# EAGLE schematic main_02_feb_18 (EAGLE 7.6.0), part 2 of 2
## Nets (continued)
Unconnected: IC1.11(CLK) IC1.18(8D) IC2.1(A:G) IC2.2(A:A1) IC2.4(A:A2) IC2.6(A:A3) IC2.8(A:A4) IC2.12(A:Y4) IC2.14(A:Y3) IC2.16(A:Y2) IC2.18(A:Y1) IC3.1(A:G) IC3.2(A:A1) IC3.4(A:A2) IC3.6(A:A3) IC3.8(A:A4) IC3.12(A:Y4) IC3.14(A:Y3) IC3.16(A:Y2) IC3.18(A:Y1) IC4.11(CLK) IC5.11(CLK) IC6.4(2D) IC6.7(3D) IC6.8(4D) IC6.11(CLK) IC6.13(5D) IC6.14(6D) IC6.17(7D) IC7.4(2D) IC7.7(3D) IC7.8(4D) IC7.13(5D) IC7.14(6D) IC7.17(7D) IC8.1(A:G) IC8.2(A:A1) IC8.4(A:A2) IC8.6(A:A3) IC8.8(A:A4) IC8.12(A:Y4) IC8.14(A:Y3) IC8.16(A:Y2) IC8.18(A:Y1) IC10.3(B:Y4) IC10.5(B:Y3) IC10.7(B:Y2) IC10.9(B:Y1) IC10.11(B:A1) IC10.13(B:A2) IC10.15(B:A3) IC10.17(B:A4) IC10.19(B:G) IC11.3(B:Y4) IC11.5(B:Y3) IC11.7(B:Y2) IC11.9(B:Y1) IC11.11(B:A1) IC11.13(B:A2) IC11.15(B:A3) IC11.17(B:A4) IC11.19(B:G) IC12.3(B:Y4) IC12.5(B:Y3) IC12.7(B:Y2) IC12.9(B:Y1) IC12.11(B:A1) IC12.13(B:A2) IC12.15(B:A3) IC12.17(B:A4) IC12.19(B:G) IC13.3(B:Y4) IC13.5(B:Y3) IC13.7(B:Y2) IC13.9(B:Y1) IC13.11(B:A1) IC13.13(B:A2) IC13.15(B:A3) IC13.17(B:A4) IC13.19(B:G) IC14.14(A=B) IC14.15(P) IC14.17(G) IC15.14(A=B) IC15.15(P) IC15.17(G) IC16.11(CLK) IC17.11(CLK) IC18.1(A:I0) IC18.2(A:I1) IC18.3(A:O) IC18.8(C:O) IC18.9(C:I0) IC18.10(C:I1) IC18.11(D:O) IC18.12(D:I0) IC18.13(D:I1) IC19.2(A:A1) IC19.4(A:A2) IC19.6(A:A3) IC19.8(A:A4) IC19.11(B:A1) IC19.13(B:A2) IC19.15(B:A3) IC19.17(B:A4) IC20.5(Q2) IC20.6(Q3) IC20.9(Q4) IC20.11(CLK) IC20.12(Q5) IC20.15(Q6) IC20.16(Q7) IC21.11(CLK) IC24.1(A:G) IC24.2(A:A1) IC24.4(A:A2) IC24.6(A:A3) IC24.8(A:A4) IC24.12(A:Y4) IC24.14(A:Y3) IC24.16(A:Y2) IC24.18(A:Y1) IC25.1(A:G) IC25.2(A:A1) IC25.4(A:A2) IC25.6(A:A3) IC25.8(A:A4) IC25.12(A:Y4) IC25.14(A:Y3) IC25.16(A:Y2) IC25.18(A:Y1) IC26.1(A:G) IC26.2(A:A1) IC26.4(A:A2) IC26.6(A:A3) IC26.8(A:A4) IC26.12(A:Y4) IC26.14(A:Y3) IC26.16(A:Y2) IC26.18(A:Y1) IC27.1(A:G) IC27.2(A:A1) IC27.4(A:A2) IC27.6(A:A3) IC27.8(A:A4) IC27.12(A:Y4) IC27.14(A:Y3) IC27.16(A:Y2) IC27.18(A:Y1) IC28.1(A:G) IC28.2(A:A1) IC28.4(A:A2) IC28.6(A:A3) IC28.8(A:A4) IC28.12(A:Y4) IC28.14(A:Y3) IC28.16(A:Y2) IC28.18(A:Y1) IC29.1(A:G) IC29.2(A:A1) IC29.4(A:A2) IC29.6(A:A3) IC29.8(A:A4) IC29.12(A:Y4) IC29.14(A:Y3) IC29.16(A:Y2) IC29.18(A:Y1) IC30.3(B:Y4) IC30.5(B:Y3) IC30.7(B:Y2) IC30.9(B:Y1) IC30.11(B:A1) IC30.13(B:A2) IC30.15(B:A3) IC30.17(B:A4) IC30.19(B:G) IC31.3(B:Y4) IC31.5(B:Y3) IC31.7(B:Y2) IC31.9(B:Y1) IC31.11(B:A1) IC31.13(B:A2) IC31.15(B:A3) IC31.17(B:A4) IC31.19(B:G) IC32.17(D7) IC32.18(D8) IC33.16(Q7) IC33.19(Q8) IC34.1(1G) IC34.15(2G) IC35.1(1G) IC35.15(2G) IC36.1(1G) IC36.15(2G) IC37.1(1G) IC37.15(2G) IC38.1(1G) IC38.15(2G) IC39.4(B:I0) IC39.5(B:I1) IC39.6(B:O) IC39.8(C:O) IC39.9(C:I0) IC39.10(C:I1) IC39.11(D:O) IC39.12(D:I0) IC39.13(D:I1) IC40.1(1G) IC40.15(2G) IC41.1(1G) IC41.15(2G) IC42.4(B:I0) IC42.5(B:I1) IC42.6(B:O) IC42.8(C:O) IC42.9(C:I0) IC42.10(C:I1) IC42.11(D:O) IC42.12(D:I0) IC42.13(D:I1) IC43.1(A:I) IC43.2(A:O) IC43.5(C:I) IC43.6(C:O) IC43.8(D:O) IC43.9(D:I) IC43.10(E:O) IC43.11(E:I) IC43.12(F:O) IC43.13(F:I) IC44.6(A:!Q) IC44.8(B:!Q) IC44.9(B:Q) IC44.10(B:PRE) IC44.11(B:CLK) IC44.12(B:D) IC44.13(B:CLR) IC45.4(B:I0) IC45.5(B:I1) IC45.6(B:O) IC45.8(C:O) IC45.9(C:I0) IC45.10(C:I1) IC45.11(D:O) IC45.12(D:I0) IC45.13(D:I1) IC46.1(G) IC46.11(CLK) IC48.4(2D) IC48.7(3D) IC48.8(4D) IC48.11(CLK) IC48.13(5D) IC48.14(6D) IC48.17(7D) IC49.3(1B) IC49.6(2B) IC49.10(3B) IC49.13(4B) IC50.1(S2) IC50.10(S4) IC50.13(S3) IC51.1(S2) IC51.4(S1) IC51.10(S4) IC51.13(S3) IC52.1(S2) IC52.4(S1) IC52.10(S4) IC52.13(S3) IC53.4(S1) IC53.9(C4) IC53.10(S4) IC53.13(S3) IC54.1(A:I) IC54.2(A:O) IC54.5(C:I) IC54.6(C:O) IC54.8(D:O) IC54.9(D:I) IC54.10(E:O) IC54.11(E:I) IC54.12(F:O) IC54.13(F:I) IC55.3(1B) IC55.6(2B) IC55.10(3B) IC56.9(2Y) IC56.10(2C0) IC56.11(2C1) IC56.12(2C2) IC56.13(2C3) IC57.5(C:I) IC57.6(C:O) IC57.8(D:O) IC57.9(D:I) IC57.10(E:O) IC57.11(E:I) IC57.12(F:O) IC57.13(F:I) IC58.4(B:I0) IC58.5(B:I1) IC58.6(B:O) IC58.8(C:O) IC58.9(C:I0) IC58.10(C:I1) IC58.11(D:O) IC58.12(D:I0) IC58.13(D:I1) IC60.1(CLR) IC60.9(Q4) IC60.12(Q5) IC60.15(Q6) IC60.16(Q7) IC60.19(Q8) IC61.1(CLR) IC61.2(Q1) IC61.5(Q2) IC61.6(Q3) IC61.9(Q4) IC61.12(Q5) IC61.15(Q6) IC61.16(Q7) IC61.19(Q8) IC62.1(CLR) IC62.2(Q1) IC62.5(Q2) IC62.6(Q3) IC62.9(Q4) IC62.12(Q5) IC62.15(Q6) IC62.16(Q7) IC62.19(Q8) IC64.8(B:O) IC64.9(B:I0) IC64.10(B:I1) IC64.12(B:I2) IC64.13(B:I3) IC65.3(B:I) IC65.4(B:O) IC65.5(C:I) IC65.6(C:O) IC65.8(D:O) IC65.9(D:I) IC65.10(E:O) IC65.11(E:I) IC65.12(F:O) IC65.13(F:I) IC66.1(A:I0) IC66.2(A:I1) IC66.3(A:O) IC66.8(C:O) IC66.9(C:I0) IC66.10(C:I1) IC66.11(D:O) IC66.12(D:I0) IC66.13(D:I1) IC67.1(A:I0) IC67.2(A:I1) IC67.3(A:O) IC67.8(C:O) IC67.9(C:I0) IC67.10(C:I1) IC67.11(D:O) IC67.12(D:I0) IC67.13(D:I1) IC68.9(3Y) IC68.12(4Y) IC69.1(A:G) IC69.2(A:A1) IC69.3(B:Y4) IC69.4(A:A2) IC69.6(A:A3) IC69.8(A:A4) IC69.12(A:Y4) IC69.14(A:Y3) IC69.15(B:A3) IC69.16(A:Y2) IC69.18(A:Y1) IC70.1(A:G) IC70.2(A:A1) IC70.4(A:A2) IC70.6(A:A3) IC70.8(A:A4) IC70.12(A:Y4) IC70.14(A:Y3) IC70.16(A:Y2) IC70.18(A:Y1) IC71.1(A:G) IC71.2(A:A1) IC71.4(A:A2) IC71.6(A:A3) IC71.8(A:A4) IC71.12(A:Y4) IC71.14(A:Y3) IC71.16(A:Y2) IC71.18(A:Y1) IC72.1(A:I0) IC72.2(A:I1) IC72.3(A:O) IC72.8(C:O) IC72.9(C:I0) IC72.10(C:I1) IC72.11(D:O) IC72.12(D:I0) IC72.13(D:I1) IC73.5(2A) IC73.6(2B) IC73.7(2Y) IC73.9(3Y) IC73.10(3B) IC73.11(3A) IC73.12(4Y) IC73.13(4B) IC73.14(4A) IC73.15(G) IC74.1(A:I0) IC74.2(A:I1) IC74.3(A:O) IC74.8(C:O) IC74.9(C:I0) IC74.10(C:I1) IC74.11(D:O) IC74.12(D:I0) IC74.13(D:I1) IC75.2(Q1) IC75.5(Q2) IC75.6(Q3) IC75.9(Q4) IC75.12(Q5) IC75.15(Q6) IC75.16(Q7) IC75.19(Q8) IC76.2(Q1) IC77.2(Q1) IC80.1(A:I0) IC80.2(A:I1) IC80.3(A:O) IC80.8(C:O) IC80.9(C:I0) IC80.10(C:I1) IC80.11(D:O) IC80.12(D:I0) IC80.13(D:I1) IC81.1(A:I0) IC81.2(A:I1) IC81.3(A:O) IC81.8(C:O) IC81.9(C:I0) IC81.10(C:I1) IC81.11(D:O) IC81.12(D:I0) IC81.13(D:I1) IC82.11(CLK) IC83.1(A:I) IC83.2(A:O) IC83.5(C:I) IC83.6(C:O) IC83.8(D:O) IC83.9(D:I) IC83.10(E:O) IC83.11(E:I) IC83.12(F:O) IC83.13(F:I) IC84.1(A:I) IC84.2(A:O) IC84.5(C:I) IC84.6(C:O) IC84.8(D:O) IC84.9(D:I) IC84.10(E:O) IC84.11(E:I) IC84.12(F:O) IC84.13(F:I) IC85.1(A:I0) IC85.2(A:I1) IC85.3(B:I0) IC85.4(B:I1) IC85.5(B:I2) IC85.6(B:O) IC85.8(C:O) IC85.9(C:I0) IC85.10(C:I1) IC85.11(C:I2) IC85.13(A:I2) IC86.11(CLK) IC87.2(A:S1) IC87.5(C:R) IC87.6(C:S) IC87.7(C:Q) IC87.9(B:Q) IC87.10(B:R) IC87.11(B:S1) IC87.12(B:S2) IC87.13(D:Q) IC87.14(D:R) IC87.15(D:S) IC88.11(CLK) IC89.3(B:Y4) IC89.5(B:Y3) IC89.7(B:Y2) IC89.9(B:Y1) IC89.11(B:A1) IC89.13(B:A2) IC89.15(B:A3) IC89.17(B:A4) IC89.19(B:G) IC90.3(B:Y4) IC90.5(B:Y3) IC90.7(B:Y2) IC90.9(B:Y1) IC90.11(B:A1) IC90.13(B:A2) IC90.15(B:A3) IC90.17(B:A4) IC90.19(B:G) IC91.3(B:Y4) IC91.5(B:Y3) IC91.7(B:Y2) IC91.9(B:Y1) IC91.11(B:A1) IC91.13(B:A2) IC91.15(B:A3) IC91.17(B:A4) IC91.19(B:G) IC92.3(B:Y4) IC92.5(B:Y3) IC92.7(B:Y2) IC92.9(B:Y1) IC92.11(B:A1) IC92.13(B:A2) IC92.15(B:A3) IC92.17(B:A4) IC92.19(B:G) IC93.11(CLK) IC98.11(CLK) IC99.11(CLK) IC100.11(CLK) IC101.11(CLK) IC102.1(A:G) IC102.2(A:A1) IC102.4(A:A2) IC102.6(A:A3) IC102.8(A:A4) IC102.12(A:Y4) IC102.14(A:Y3) IC102.16(A:Y2) IC102.18(A:Y1) IC103.12(Y7) IC103.13(Y6) IC103.15(Y4) IC103.16(Y3) IC103.17(Y2) IC104.12(Y7) IC104.13(Y6) IC104.14(Y5) IC104.15(Y4) IC104.16(Y3) IC105.1(A:G) IC105.2(A:A1) IC105.4(A:A2) IC105.6(A:A3) IC105.8(A:A4) IC105.12(A:Y4) IC105.14(A:Y3) IC105.16(A:Y2) IC105.18(A:Y1) IC106.1(A:G) IC106.2(A:A1) IC106.4(A:A2) IC106.6(A:A3) IC106.8(A:A4) IC106.12(A:Y4) IC106.14(A:Y3) IC106.16(A:Y2) IC106.18(A:Y1) IC107.1(A:G) IC107.2(A:A1) IC107.4(A:A2) IC107.6(A:A3) IC107.8(A:A4) IC107.12(A:Y4) IC107.14(A:Y3) IC107.16(A:Y2) IC107.18(A:Y1) IC108.1(A:G) IC108.2(A:A1) IC108.4(A:A2) IC108.6(A:A3) IC108.8(A:A4) IC108.12(A:Y4) IC108.14(A:Y3) IC108.16(A:Y2) IC108.18(A:Y1) IC109.1(A:G) IC109.2(A:A1) IC109.4(A:A2) IC109.6(A:A3) IC109.8(A:A4) IC109.12(A:Y4) IC109.14(A:Y3) IC109.16(A:Y2) IC109.18(A:Y1) IC110.1(A:G) IC110.2(A:A1) IC110.4(A:A2) IC110.6(A:A3) IC110.8(A:A4) IC110.12(A:Y4) IC110.14(A:Y3) IC110.16(A:Y2) IC110.18(A:Y1) IC111.1(A:G) IC111.2(A:A1) IC111.4(A:A2) IC111.6(A:A3) IC111.8(A:A4) IC111.12(A:Y4) IC111.14(A:Y3) IC111.16(A:Y2) IC111.18(A:Y1) IC112.1(A:G) IC112.2(A:A1) IC112.4(A:A2) IC112.6(A:A3) IC112.8(A:A4) IC112.12(A:Y4) IC112.14(A:Y3) IC112.16(A:Y2) IC112.18(A:Y1) IC113.1(A:G) IC113.2(A:A1) IC113.4(A:A2) IC113.6(A:A3) IC113.8(A:A4) IC113.12(A:Y4) IC113.14(A:Y3) IC113.16(A:Y2) IC113.18(A:Y1) IC114.1(A:G) IC114.2(A:A1) IC114.4(A:A2) IC114.6(A:A3) IC114.8(A:A4) IC114.12(A:Y4) IC114.14(A:Y3) IC114.16(A:Y2) IC114.18(A:Y1) IC115.1(A:G) IC115.2(A:A1) IC115.4(A:A2) IC115.6(A:A3) IC115.8(A:A4) IC115.12(A:Y4) IC115.14(A:Y3) IC115.16(A:Y2) IC115.18(A:Y1) IC116.1(A:G) IC116.2(A:A1) IC116.4(A:A2) IC116.6(A:A3) IC116.8(A:A4) IC116.12(A:Y4) IC116.14(A:Y3) IC116.16(A:Y2) IC116.18(A:Y1) IC117.1(A:G) IC117.2(A:A1) IC117.4(A:A2) IC117.6(A:A3) IC117.8(A:A4) IC117.12(A:Y4) IC117.14(A:Y3) IC117.16(A:Y2) IC117.18(A:Y1) IC118.1(G1) IC118.11(Y8) IC118.12(Y7) IC118.19(G2) IC119.5(2A) IC119.6(2B) IC119.7(2Y) IC119.9(3Y) IC119.10(3B) IC119.11(3A) IC119.12(4Y) IC119.13(4B) IC119.14(4A) IC120.4(B:I0) IC120.5(B:I1) IC120.6(B:O) IC120.8(C:O) IC120.9(C:I0) IC120.10(C:I1) IC120.11(D:O) IC120.12(D:I0) IC120.13(D:I1) IC121.5(2A) IC121.6(2B) IC121.7(2Y) IC121.9(3Y) IC121.10(3B) IC121.11(3A) IC121.12(4Y) IC121.13(4B) IC121.14(4A) IC123.11(CLK) IC123.18(8D) IC124.1(A:G) IC124.2(A:A1) IC124.4(A:A2) IC124.6(A:A3) IC124.8(A:A4) IC124.12(A:Y4) IC124.14(A:Y3) IC124.16(A:Y2) IC124.18(A:Y1) IC125.1(A:G) IC125.2(A:A1) IC125.4(A:A2) IC125.6(A:A3) IC125.8(A:A4) IC125.12(A:Y4) IC125.14(A:Y3) IC125.16(A:Y2) IC125.18(A:Y1) IC126.11(CLK) IC126.12(5Q) IC126.13(5D) IC126.14(6D) IC126.15(6Q) IC126.16(7Q) IC126.17(7D) IC126.18(8D) IC126.19(8Q) IC127.4(B:I0) IC127.5(B:I1) IC127.6(B:O) IC127.8(C:O) IC127.9(C:I0) IC127.10(C:I1) IC127.11(D:O) IC127.12(D:I0) IC127.13(D:I1) IC129.1(A:G) IC129.2(A:A1) IC129.4(A:A2) IC129.6(A:A3) IC129.8(A:A4) IC129.12(A:Y4) IC129.14(A:Y3) IC129.16(A:Y2) IC129.18(A:Y1) IC130.1(A:I0) IC130.2(A:I1) IC130.3(A:O) IC130.8(C:O) IC130.9(C:I0) IC130.10(C:I1) IC130.11(D:O) IC130.12(D:I0) IC130.13(D:I1) IC131.8(B:O) IC131.9(B:I0) IC131.10(B:I1) IC131.12(B:I2) IC131.13(B:I3) IC132.3(B:I) IC132.4(B:O) IC132.5(C:I) IC132.6(C:O) IC132.8(D:O) IC132.9(D:I) IC132.10(E:O) IC132.11(E:I) IC132.12(F:O) IC132.13(F:I) IC133.3(A:O) IC133.4(B:I0) IC133.5(B:I1) IC133.6(B:O) IC133.8(C:O) IC133.9(C:I0) IC133.10(C:I1) IC133.11(D:O) IC133.12(D:I0) IC133.13(D:I1) IC138.4(B:I0) IC138.5(B:I1) IC138.6(B:O) IC138.8(C:O) IC138.9(C:I0) IC138.10(C:I1) IC138.11(D:O) IC138.12(D:I0) IC138.13(D:I1) IC139.4(Q2) IC139.5(Q3) IC139.6(Q4) IC139.11(D4) IC139.12(D3) IC139.13(D2) IC140.1(G1) IC140.19(G2) IC141.3(B:I) IC141.4(B:O) IC141.5(C:I) IC141.6(C:O) IC141.8(D:O) IC141.9(D:I) IC141.10(E:O) IC141.11(E:I) IC141.12(F:O) IC141.13(F:I) IC142.1(1G) IC142.15(2G) IC143.4(B:I0) IC143.5(B:I1) IC143.6(B:O) IC143.8(C:O) IC143.9(C:I0) IC143.10(C:I1) IC143.11(D:O) IC143.12(D:I0) IC143.13(D:I1) IC145.1(A:G) IC145.2(A:A1) IC145.4(A:A2) IC145.6(A:A3) IC145.8(A:A4) IC145.12(A:Y4) IC145.14(A:Y3) IC145.16(A:Y2) IC145.18(A:Y1) IC146.1(A:G) IC146.2(A:A1) IC146.4(A:A2) IC146.6(A:A3) IC146.8(A:A4) IC146.12(A:Y4) IC146.14(A:Y3) IC146.16(A:Y2) IC146.18(A:Y1) IC147.1(A:I0) IC147.2(A:I1) IC147.3(A:O) IC147.8(C:O) IC147.9(C:I0) IC147.10(C:I1) IC147.11(D:O) IC147.12(D:I0) IC147.13(D:I1) IC148.1(A:I) IC148.2(A:O) IC148.5(C:I) IC148.6(C:O) IC148.8(D:O) IC148.9(D:I) IC148.10(E:O) IC148.11(E:I) IC148.12(F:O) IC148.13(F:I) IC149.1(A:I) IC149.2(A:O) IC149.5(C:I) IC149.6(C:O) IC149.8(D:O) IC149.9(D:I) IC149.10(E:O) IC149.11(E:I) IC149.12(F:O) IC149.13(F:I) IC150.3(B:I) IC150.4(B:O) IC150.5(C:I) IC150.6(C:O) IC150.8(D:O) IC150.9(D:I) IC150.10(E:O) IC150.11(E:I) IC150.12(F:O) IC150.13(F:I) IC151.3(B:I) IC151.4(B:O) IC151.5(C:I) IC151.6(C:O) IC151.8(D:O) IC151.9(D:I) IC151.10(E:O) IC151.11(E:I) IC151.12(F:O) IC151.13(F:I) IC152.1(A:I) IC152.2(A:O) IC152.5(C:I) IC152.6(C:O) IC152.8(D:O) IC152.9(D:I) IC152.10(E:O) IC152.11(E:I) IC152.12(F:O) IC152.13(F:I) IC153.11(CLK) IC154.1(A:G) IC154.2(A:A1) IC154.4(A:A2) IC154.6(A:A3) IC154.8(A:A4) IC154.12(A:Y4) IC154.14(A:Y3) IC154.16(A:Y2) IC154.18(A:Y1) IC155.1(A:G) IC155.2(A:A1) IC155.4(A:A2) IC155.6(A:A3) IC155.8(A:A4) IC155.12(A:Y4) IC155.14(A:Y3) IC155.16(A:Y2) IC155.18(A:Y1) IC156.1(A:G) IC156.2(A:A1) IC156.4(A:A2) IC156.6(A:A3) IC156.8(A:A4) IC156.12(A:Y4) IC156.14(A:Y3) IC156.16(A:Y2) IC156.18(A:Y1) IC157.3(B:I) IC157.4(B:O) IC157.5(C:I) IC157.6(C:O) IC157.8(D:O) IC157.9(D:I) IC157.10(E:O) IC157.11(E:I) IC157.12(F:O) IC157.13(F:I) IC158.3(B:I) IC158.4(B:O) IC158.5(C:I) IC158.6(C:O) IC158.8(D:O) IC158.9(D:I) IC158.10(E:O) IC158.11(E:I) IC158.12(F:O) IC158.13(F:I) IC159.1(A:G) IC159.2(A:A1) IC159.4(A:A2) IC159.6(A:A3) IC159.8(A:A4) IC159.12(A:Y4) IC159.14(A:Y3) IC159.16(A:Y2) IC159.18(A:Y1) IC160.1(A:G) IC160.2(A:A1) IC160.4(A:A2) IC160.6(A:A3) IC160.8(A:A4) IC160.12(A:Y4) IC160.14(A:Y3) IC160.16(A:Y2) IC160.18(A:Y1) IC161.1(A:G) IC161.2(A:A1) IC161.4(A:A2) IC161.6(A:A3) IC161.8(A:A4) IC161.12(A:Y4) IC161.14(A:Y3) IC161.16(A:Y2) IC161.18(A:Y1) IC163.6(A:!Q) IC163.8(B:!Q) IC163.9(B:Q) IC163.10(B:PRE) IC163.11(B:CLK) IC163.12(B:D) IC163.13(B:CLR) IC164.6(A:!Q) IC164.8(B:!Q) IC164.9(B:Q) IC164.10(B:PRE) IC164.11(B:CLK) IC164.12(B:D) IC164.13(B:CLR) IC165.1(G1) IC165.2(A1) IC165.3(A2) IC165.4(A3) IC165.5(A4) IC165.6(A5) IC165.7(A6) IC165.8(A7) IC165.9(A8) IC165.11(Y8) IC165.12(Y7) IC165.14(Y5) IC165.15(Y4) IC165.16(Y3) IC165.17(Y2) IC165.18(Y1) IC165.19(G2) IC166.1(G1) IC166.4(A3) IC166.5(A4) IC166.6(A5) IC166.7(A6) IC166.8(A7) IC166.9(A8) IC166.11(Y8) IC166.12(Y7) IC166.13(Y6) IC166.14(Y5) IC166.15(Y4) IC166.16(Y3) IC166.19(G2) IC167.5(2A) IC167.6(2B) IC167.7(2Y) IC167.9(3Y) IC167.10(3B) IC167.11(3A) IC167.12(4Y) IC167.13(4B) IC167.14(4A) IC168.6(A:!Q) IC168.8(B:!Q) IC168.9(B:Q) IC168.10(B:PRE) IC168.11(B:CLK) IC168.12(B:D) IC168.13(B:CLR) IC169.15(G) IC170.1(A:I0) IC170.2(A:I1) IC170.3(A:O) IC170.8(C:O) IC170.9(C:I0) IC170.10(C:I1) IC170.11(D:O) IC170.12(D:I0) IC170.13(D:I1) IC171.15(G) IC172.9(3Y) IC172.12(4Y) IC172.15(G) IC173.15(G) IC174.6(A:!Q) IC174.8(B:!Q) IC174.9(B:Q) IC174.10(B:PRE) IC174.11(B:CLK) IC174.12(B:D) IC174.13(B:CLR) IC175.1(A:I0) IC175.2(A:I1) IC175.3(A:O) IC175.8(C:O) IC175.9(C:I0) IC175.10(C:I1) IC175.11(D:O) IC175.12(D:I0) IC175.13(D:I1) IC176.3(B:Y4) IC176.5(B:Y3) IC176.7(B:Y2) IC176.9(B:Y1) IC176.11(B:A1) IC176.13(B:A2) IC176.15(B:A3) IC176.17(B:A4) IC176.19(B:G) IC177.1(A:I0) IC177.2(A:I1) IC177.3(A:O) IC177.8(C:O) IC177.9(C:I0) IC177.10(C:I1) IC177.11(D:O) IC177.12(D:I0) IC177.13(D:I1) IC178.3(B:Y4) IC178.5(B:Y3) IC178.7(B:Y2) IC178.9(B:Y1) IC178.11(B:A1) IC178.13(B:A2) IC178.15(B:A3) IC178.17(B:A4) IC178.19(B:G) IC179.3(B:Y4) IC179.5(B:Y3) IC179.7(B:Y2) IC179.9(B:Y1) IC179.11(B:A1) IC179.13(B:A2) IC179.15(B:A3) IC179.17(B:A4) IC179.19(B:G) IC180.11(CLK) IC181.3(B:Y4) IC181.5(B:Y3) IC181.7(B:Y2) IC181.9(B:Y1) IC181.11(B:A1) IC181.13(B:A2) IC181.15(B:A3) IC181.17(B:A4) IC181.19(B:G) IC182.3(B:Y4) IC182.5(B:Y3) IC182.7(B:Y2) IC182.9(B:Y1) IC182.11(B:A1) IC182.13(B:A2) IC182.15(B:A3) IC182.17(B:A4) IC182.19(B:G) IC183.3(B:Y4) IC183.5(B:Y3) IC183.7(B:Y2) IC183.9(B:Y1) IC183.11(B:A1) IC183.13(B:A2) IC183.15(B:A3) IC183.17(B:A4) IC183.19(B:G) IC184.11(CLK) IC185.11(CLK) IC186.1(A:G) IC186.2(A:A1) IC186.4(A:A2) IC186.6(A:A3) IC186.8(A:A4) IC186.12(A:Y4) IC186.14(A:Y3) IC186.16(A:Y2) IC186.18(A:Y1) IC187.6(A:!Q) IC187.8(B:!Q) IC187.9(B:Q) IC187.10(B:PRE) IC187.11(B:CLK) IC187.12(B:D) IC187.13(B:CLR) IC188.6(A:!Q) IC188.8(B:!Q) IC188.9(B:Q) IC188.10(B:PRE) IC188.11(B:CLK) IC188.12(B:D) IC188.13(B:CLR) IC189.4(2D) IC189.7(3D) IC189.8(4D) IC189.13(5D) IC189.14(6D) IC189.17(7D) IC190.1(A:I0) IC190.2(A:I1) IC190.3(A:O) IC190.4(B:I0) IC190.5(B:I1) IC190.6(B:O) IC190.11(D:O) IC190.12(D:I0) IC190.13(D:I1) IC191.4(B:I0) IC191.5(B:I1) IC191.6(B:O) IC191.8(C:O) IC191.9(C:I0) IC191.10(C:I1) IC191.11(D:O) IC191.12(D:I0) IC191.13(D:I1) IC192.1(A:I0) IC192.2(A:I1) IC192.3(A:O) IC192.8(C:O) IC192.9(C:I0) IC192.10(C:I1) IC192.11(D:O) IC192.12(D:I0) IC192.13(D:I1) IC193.1(A:I0) IC193.2(A:I1) IC193.3(A:O) IC193.8(C:O) IC193.9(C:I0) IC193.10(C:I1) IC193.11(D:O) IC193.12(D:I0) IC193.13(D:I1) IC194.1(A:I0) IC194.2(A:I1) IC194.3(A:O) IC194.8(C:O) IC194.9(C:I0) IC194.10(C:I1) IC194.11(D:O) IC194.12(D:I0) IC194.13(D:I1) IC195.1(A:G) IC195.2(A:A1) IC195.4(A:A2) IC195.6(A:A3) IC195.8(A:A4) IC195.12(A:Y4) IC195.14(A:Y3) IC195.16(A:Y2) IC195.18(A:Y1) IC196.1(A:G) IC196.2(A:A1) IC196.4(A:A2) IC196.6(A:A3) IC196.8(A:A4) IC196.12(A:Y4) IC196.14(A:Y3) IC196.16(A:Y2) IC196.18(A:Y1) IC197.4(B:I0) IC197.6(B:O) IC197.8(B:I1) IC197.9(B:I2) IC197.10(B:I3) IC197.11(B:I4) IC198.3(B:I) IC198.4(B:O) IC198.5(C:I) IC198.6(C:O) IC198.8(D:O) IC198.9(D:I) IC198.10(E:O) IC198.11(E:I) IC198.12(F:O) IC198.13(F:I) IC199.4(B:I0) IC199.6(B:O) IC199.8(B:I1) IC199.9(B:I2) IC199.10(B:I3) IC199.11(B:I4) IC200.1(A:I0) IC200.2(A:I1) IC200.3(A:O) IC200.8(C:O) IC200.9(C:I0) IC200.10(C:I1) IC200.11(D:O) IC200.12(D:I0) IC200.13(D:I1) IC201.1(A:I0) IC201.2(A:I1) IC201.3(A:O) IC201.4(B:I0) IC201.5(B:I1) IC201.6(B:O) IC201.11(D:O) IC201.12(D:I0) IC201.13(D:I1) IC202.4(B:I0) IC202.5(B:I1) IC202.6(B:O) IC202.8(C:O) IC202.9(C:I0) IC202.10(C:I1) IC202.11(D:O) IC202.12(D:I0) IC202.13(D:I1) IC203.1(A:I0) IC203.2(A:I1) IC203.3(A:O) IC203.4(B:I0) IC203.5(B:I1) IC203.6(B:O) IC203.11(D:O) IC203.12(D:I0) IC203.13(D:I1) IC204.3(B:I0) IC204.4(B:I1) IC204.5(B:I2) IC204.6(B:O) IC204.8(C:O) IC204.9(C:I0) IC204.10(C:I1) IC204.11(C:I2) IC205.4(B:I0) IC205.5(B:I1) IC205.6(B:O) IC205.8(C:O) IC205.9(C:I0) IC205.10(C:I1) IC205.11(D:O) IC205.12(D:I0) IC205.13(D:I1) IC206.1(A:I0) IC206.2(A:I1) IC206.3(A:O) IC206.4(B:I0) IC206.5(B:I1) IC206.6(B:O) IC206.11(D:O) IC206.12(D:I0) IC206.13(D:I1) IC207.4(B:I0) IC207.5(B:I1) IC207.6(B:O) IC207.8(C:O) IC207.9(C:I0) IC207.10(C:I1) IC207.11(D:O) IC207.12(D:I0) IC207.13(D:I1) IC208.4(B:I0) IC208.5(B:I1) IC208.6(B:O) IC208.8(C:O) IC208.9(C:I0) IC208.10(C:I1) IC208.11(D:O) IC208.12(D:I0) IC208.13(D:I1) IC209.1(A:I0) IC209.2(A:I1) IC209.3(A:O) IC209.8(C:O) IC209.9(C:I0) IC209.10(C:I1) IC209.11(D:O) IC209.12(D:I0) IC209.13(D:I1) IC211.3(B:Y4) IC211.5(B:Y3) IC211.7(B:Y2) IC211.9(B:Y1) IC211.11(B:A1) IC211.13(B:A2) IC211.15(B:A3) IC211.17(B:A4) IC211.19(B:G) IC212.3(B:Y4) IC212.5(B:Y3) IC212.7(B:Y2) IC212.9(B:Y1) IC212.11(B:A1) IC212.13(B:A2) IC212.15(B:A3) IC212.17(B:A4) IC212.19(B:G) IC213.3(B:Y4) IC213.5(B:Y3) IC213.7(B:Y2) IC213.9(B:Y1) IC213.11(B:A1) IC213.13(B:A2) IC213.15(B:A3) IC213.17(B:A4) IC213.19(B:G) IC214.3(B:Y4) IC214.5(B:Y3) IC214.7(B:Y2) IC214.9(B:Y1) IC214.11(B:A1) IC214.13(B:A2) IC214.15(B:A3) IC214.17(B:A4) IC214.19(B:G) IC215.1(A:G) IC215.2(A:A1) IC215.4(A:A2) IC215.6(A:A3) IC215.8(A:A4) IC215.12(A:Y4) IC215.14(A:Y3) IC215.16(A:Y2) IC215.18(A:Y1) IC216.1(G) IC216.11(CLK) IC218.4(B:I0) IC218.5(B:I1) IC218.6(B:O) IC218.8(C:O) IC218.9(C:I0) IC218.10(C:I1) IC218.11(D:O) IC218.12(D:I0) IC218.13(D:I1) IC219.4(B:I0) IC219.5(B:I1) IC219.6(B:O) IC219.8(C:O) IC219.9(C:I0) IC219.10(C:I1) IC219.11(D:O) IC219.12(D:I0) IC219.13(D:I1) IC220.4(B:I0) IC220.5(B:I1) IC220.6(B:O) IC220.8(C:O) IC220.9(C:I0) IC220.10(C:I1) IC220.11(D:O) IC220.12(D:I0) IC220.13(D:I1) IC221.6(A:!Q) IC221.8(B:!Q) IC221.9(B:Q) IC221.10(B:PRE) IC221.11(B:CLK) IC221.12(B:D) IC221.13(B:CLR) IC222.14(Y1) IC223.4(B:I0) IC223.5(B:I1) IC223.6(B:O) IC223.8(C:O) IC223.9(C:I0) IC223.10(C:I1) IC223.11(D:O) IC223.12(D:I0) IC223.13(D:I1) IC224.4(B:I0) IC224.5(B:I1) IC224.6(B:O) IC224.8(C:O) IC224.9(C:I0) IC224.10(C:I1) IC224.11(D:O) IC224.12(D:I0) IC224.13(D:I1) IC225.4(B:I0) IC225.5(B:I1) IC225.6(B:O) IC225.8(C:O) IC225.9(C:I0) IC225.10(C:I1) IC225.11(D:O) IC225.12(D:I0) IC225.13(D:I1) IC227.4(B:I0) IC227.5(B:I1) IC227.6(B:O) IC227.8(C:O) IC227.9(C:I0) IC227.10(C:I1) IC227.11(D:O) IC227.12(D:I0) IC227.13(D:I1) IC228.1(A:I0) IC228.2(A:I1) IC228.3(A:O) IC228.4(B:I0) IC228.5(B:I1) IC228.6(B:O) IC228.11(D:O) IC228.12(D:I0) IC228.13(D:I1) IC229.3(B:Y4) IC229.5(B:Y3) IC229.7(B:Y2) IC229.9(B:Y1) IC229.11(B:A1) IC229.13(B:A2) IC229.15(B:A3) IC229.17(B:A4) IC229.19(B:G) IC230.3(B:Y4) IC230.5(B:Y3) IC230.7(B:Y2) IC230.9(B:Y1) IC230.11(B:A1) IC230.13(B:A2) IC230.15(B:A3) IC230.17(B:A4) IC230.19(B:G) IC231.3(B:Y4) IC231.5(B:Y3) IC231.7(B:Y2) IC231.9(B:Y1) IC231.11(B:A1) IC231.13(B:A2) IC231.15(B:A3) IC231.17(B:A4) IC231.19(B:G) IC232.3(B:Y4) IC232.5(B:Y3) IC232.7(B:Y2) IC232.9(B:Y1) IC232.11(B:A1) IC232.13(B:A2) IC232.15(B:A3) IC232.17(B:A4) IC232.19(B:G) IC233.11(CLK) IC234.11(CLK) IC235.3(B:Y4) IC235.5(B:Y3) IC235.7(B:Y2) IC235.9(B:Y1) IC235.11(B:A1) IC235.13(B:A2) IC235.15(B:A3) IC235.17(B:A4) IC235.19(B:G) IC236.3(B:Y4) IC236.5(B:Y3) IC236.7(B:Y2) IC236.9(B:Y1) IC236.11(B:A1) IC236.13(B:A2) IC236.15(B:A3) IC236.17(B:A4) IC236.19(B:G) IC237.3(B:Y4) IC237.5(B:Y3) IC237.7(B:Y2) IC237.9(B:Y1) IC237.11(B:A1) IC237.13(B:A2) IC237.15(B:A3) IC237.17(B:A4) IC237.19(B:G) IC238.3(B:Y4) IC238.5(B:Y3) IC238.7(B:Y2) IC238.9(B:Y1) IC238.11(B:A1) IC238.13(B:A2) IC238.15(B:A3) IC238.17(B:A4) IC238.19(B:G) IC239.11(CLK) IC240.11(CLK) IC241.4(B:I0) IC241.5(B:I1) IC241.6(B:O) IC241.8(C:O) IC241.9(C:I0) IC241.10(C:I1) IC241.11(D:O) IC241.12(D:I0) IC241.13(D:I1) IC242.1(A:I0) IC242.2(A:I1) IC242.3(A:O) IC242.4(B:I0) IC242.5(B:I1) IC242.6(B:O) IC242.11(D:O) IC242.12(D:I0) IC242.13(D:I1) IC243.4(B:I0) IC243.5(B:I1) IC243.6(B:O) IC243.8(C:O) IC243.9(C:I0) IC243.10(C:I1) IC243.11(D:O) IC243.12(D:I0) IC243.13(D:I1) IC244.1(A:G) IC244.2(A:A1) IC244.4(A:A2) IC244.6(A:A3) IC244.8(A:A4) IC244.12(A:Y4) IC244.14(A:Y3) IC244.16(A:Y2) IC244.18(A:Y1) IC245.3(B:Y4) IC245.5(B:Y3) IC245.7(B:Y2) IC245.9(B:Y1) IC245.11(B:A1) IC245.13(B:A2) IC245.15(B:A3) IC245.17(B:A4) IC245.19(B:G) IC246.3(B:Y4) IC246.5(B:Y3) IC246.7(B:Y2) IC246.9(B:Y1) IC246.11(B:A1) IC246.13(B:A2) IC246.15(B:A3) IC246.17(B:A4) IC246.19(B:G) IC247.1(A:G) IC247.2(A:A1) IC247.4(A:A2) IC247.6(A:A3) IC247.8(A:A4) IC247.12(A:Y4) IC247.14(A:Y3) IC247.16(A:Y2) IC247.18(A:Y1) IC250.1(A:I0) IC250.2(A:I1) IC250.3(A:O) IC250.8(C:O) IC250.9(C:I0) IC250.10(C:I1) IC250.11(D:O) IC250.12(D:I0) IC250.13(D:I1) R10.1 R10.2 R10.3 R10.4 R10.5 R10.12 R10.13 R10.14 R10.15 R10.16 S2.1(O) S3.1 S3.2 S3.3 S3.4 S3.5 S3.6 S3.7 S3.8 S3.9 S3.10 S3.11 S3.12 S3.13 S3.14 S3.15 S3.16 S3.C1(C) S4.1(O) SW3.8 U$1.28(VCC) U$2.28(VCC) U$3.28(VCC) U$4.28(VCC) U$5.28(VCC) U$6.28(VCC) U$7.28(VCC) U$8.28(VCC) U$9.28(VCC) U$10.1(A14) U$10.2(A12) U$10.3(A7) U$10.4(A6) U$10.5(A5) U$10.6(A4) U$10.7(A3) U$10.8(A2) U$10.9(A1) U$10.10(A0) U$10.14(GND) U$10.20(/CE) U$10.21(A10) U$10.22(/OE) U$10.23(A11) U$10.24(A9) U$10.25(A8) U$10.26(A13) U$10.27(/WE) U$10.28(VCC) U$11.1(A14) U$11.2(A12) U$11.3(A7) U$11.4(A6) U$11.5(A5) U$11.6(A4) U$11.7(A3) U$11.8(A2) U$11.9(A1) U$11.10(A0) U$11.14(GND) U$11.20(/CE) U$11.21(A10) U$11.22(/OE) U$11.23(A11) U$11.24(A9) U$11.25(A8) U$11.26(A13) U$11.27(/WE) U$11.28(VCC) U$12.1(A14) U$12.2(A12) U$12.3(A7) U$12.4(A6) U$12.5(A5) U$12.6(A4) U$12.7(A3) U$12.8(A2) U$12.9(A1) U$12.10(A0) U$12.14(GND) U$12.20(/CE) U$12.21(A10) U$12.22(/OE) U$12.23(A11) U$12.24(A9) U$12.25(A8) U$12.26(A13) U$12.27(/WE) U$12.28(VCC)

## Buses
XBUS[0..7]
ZBUS[0..7]
YBUS[0..7]
AD[0..15]
MDR_IN_BUS[0..7]
U_AD[0..13]
DATA[0..7]
U_AD_BUFF[0..13]
Z_BUS[0..7]
U_ADDR_BUFF1_[0..13]

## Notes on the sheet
- TRAP
  DMA_REQ
  INT_REQ_0
  INT_REQ_1
  INT_REQ_2
  INT_REQ_3
  INT_REQ_4
  INT_REQ_5
- might need to flip flop this output in case it oscillates
- SYNCHRONIZED INTERRUPT INPUTS
- trap = 000
  dma = 001
  
  there will be a hole in memory in the interrupt
  vector because dma is between trap and 
  the other interrupts.
- SINGLE STEP CLOCK
- IMMX
- fast clock
- slow clock
- TDR0_L
- TDR0_H
- TDR1_L
- TDR1_H
- MASK_FLAGS
- R_SHIFT_L
- U-ADDRESS MUX
- R_SHIFT_H
- OFFSET(6)
- AL
- Z BUS
- PC_L
- U-CODE ROMS
- U-ADDRESS
- IR | U-CODE FF'S
- AH
- ADDRESS & DATA BUSES NEED PULL DOWN RESISTORS 
  BECAUSE THE CPU BUS OUTPUTS HAVE 
  244'S WHICH ARE CLOSED MOST OF THE TIME.
- LOW | ADDRESS BUS | PC_H
- MARL
- LOW
- ADDER
- BL
- HIGH
- SP_L
- BH
- ADDER
- MARH
- MAR is tri-stated when in programming or DMA mode. | SP_H
- programming mode signal goes here to tell MAR to go tristate
- CL
- AUX_FLAGS
- U-CODE FF'S
- BP_L
- CH
- if type = branch, and condition = false, then next = +1
- HIGH
- BP_H
- DL
- U-ADDRESS MUX
- Z BUS
- MUX1
- DH
- U_FLAGS
- CARRY IN MUX
- CONDITION SOURCE
  PROGRAMMER'S FLAGS 
  OR
  U_CODE FLAGS
- DATA BUS
- ZF
- BUS GOING INTO MDR INPUTS
- CF / LTU
- SF
- OF
- BUS GOING INTO MDR INPUTS
- PF
- X BUS
- LT
  LTE
  ~LT = GTE
  ~LTE + GT
- MDR_L
- IMMY | MDR MUX
- MDR_H
- ALU
- alu_mode removed. OF is undefined if alu in logic mode anyway. | alu_op == add
- DATA BUS
- ALU_OP == SUB
- TDR0_L
- IMMY
- TDR0_H
- FROM MICROCODE
- TDR1_L
- TDR1_H
- THESE TDR'S ARE THE SAME ONES AS ARE CONNECTED TO THE X BUS

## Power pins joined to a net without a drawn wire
GND: IC1.10(GND) IC2.10(P:GND) IC3.10(P:GND) IC4.10(GND) IC5.10(GND) IC6.10(GND) IC7.10(GND) IC8.10(P:GND) IC9.10(P:GND) IC10.10(P:GND) IC11.10(P:GND) IC12.10(P:GND) IC13.10(P:GND) IC14.12(GND) IC15.12(GND) IC16.10(GND) IC17.10(GND) IC18.7(P:GND) IC19.10(P:GND) IC20.10(GND) IC21.10(GND) IC22.8(GND) IC23.8(GND) IC24.10(P:GND) IC25.10(P:GND) IC26.10(P:GND) IC27.10(P:GND) IC28.10(P:GND) IC29.10(P:GND) IC30.10(P:GND) IC31.10(P:GND) IC32.10(GND) IC33.10(GND) IC34.8(GND) IC35.8(GND) IC36.8(GND) IC37.8(GND) IC38.8(GND) IC39.7(P:GND) IC40.8(GND) IC41.8(GND) IC42.7(P:GND) IC43.7(P:GND) IC44.7(P:GND) IC45.7(P:GND) IC46.10(GND) IC47.8(GND) IC48.10(GND) IC49.8(GND) IC50.8(GND) IC51.8(GND) IC52.8(GND) IC53.8(GND) IC54.7(P:GND) IC55.8(GND) IC56.8(GND) IC57.7(P:GND) IC58.7(P:GND) IC59.8(GND) IC60.10(GND) IC61.10(GND) IC62.10(GND) IC63.8(GND) IC64.7(P:GND) IC65.7(P:GND) IC66.7(P:GND) IC67.7(P:GND) IC68.8(GND) IC69.10(P:GND) IC70.10(P:GND) IC71.10(P:GND) IC72.7(P:GND) IC73.8(GND) IC74.7(P:GND) IC75.10(GND) IC76.10(GND) IC77.10(GND) IC78.10(GND) IC79.10(GND) IC80.7(P:GND) IC81.7(P:GND) IC82.10(GND) IC83.7(P:GND) IC84.7(P:GND) IC85.7(P:GND) IC86.10(GND) IC87.8(P:GND) IC88.10(GND) IC89.10(P:GND) IC90.10(P:GND) IC91.10(P:GND) IC92.10(P:GND) IC93.10(GND) IC94.8(GND) IC95.8(GND) IC96.8(GND) IC97.8(GND) IC98.10(GND) IC99.10(GND) IC100.10(GND) IC101.10(GND) IC102.10(P:GND) IC103.10(GND) IC104.10(GND) IC105.10(P:GND) IC106.10(P:GND) IC107.10(P:GND) IC108.10(P:GND) IC109.10(P:GND) IC110.10(P:GND) IC111.10(P:GND) IC112.10(P:GND) IC113.10(P:GND) IC114.10(P:GND) IC115.10(P:GND) IC116.10(P:GND) IC117.10(P:GND) IC118.10(GND) IC119.8(GND) IC120.7(P:GND) IC121.8(GND) IC122.10(P:GND) IC123.10(GND) IC124.10(P:GND) IC125.10(P:GND) IC126.10(GND) IC127.7(P:GND) IC128.8(GND) IC129.10(P:GND) IC130.7(P:GND) IC131.7(P:GND) IC132.7(P:GND) IC133.7(P:GND) IC134.10(GND) IC135.10(GND) IC136.10(GND) IC137.10(GND) IC138.7(P:GND) IC139.8(GND) IC140.10(GND) IC141.7(P:GND) IC142.8(GND) IC143.7(P:GND) IC144.8(GND) IC145.10(P:GND) IC146.10(P:GND) IC147.7(P:GND) IC148.7(P:GND) IC149.7(P:GND) IC150.7(P:GND) IC151.7(P:GND) IC152.7(P:GND) IC153.10(GND) IC154.10(P:GND) IC155.10(P:GND) IC156.10(P:GND) IC157.7(P:GND) IC158.7(P:GND) IC159.10(P:GND) IC160.10(P:GND) IC161.10(P:GND) IC162.10(GND) IC163.7(P:GND) IC164.7(P:GND) IC165.10(GND) IC166.10(GND) IC167.8(GND) IC168.7(P:GND) IC169.8(GND) IC170.7(P:GND) IC171.8(GND) IC172.8(GND) IC173.8(GND) IC174.7(P:GND) IC175.7(P:GND) IC176.10(P:GND) IC177.7(P:GND) IC178.10(P:GND) IC179.10(P:GND) IC180.10(GND) IC181.10(P:GND) IC182.10(P:GND) IC183.10(P:GND) IC184.10(GND) IC185.10(GND) IC186.10(P:GND) IC187.7(P:GND) IC188.7(P:GND) IC189.10(GND) IC190.7(P:GND) IC191.7(P:GND) IC192.7(P:GND) IC193.7(P:GND) IC194.7(P:GND) IC195.10(P:GND) IC196.10(P:GND) IC197.7(P:GND) IC198.7(P:GND) IC199.7(P:GND) IC200.7(P:GND) IC201.7(P:GND) IC202.7(P:GND) IC203.7(P:GND) IC204.7(P:GND) IC205.7(P:GND) IC206.7(P:GND) IC207.7(P:GND) IC208.7(P:GND) IC209.7(P:GND) IC210.8(GND) IC211.10(P:GND) IC212.10(P:GND) IC213.10(P:GND) IC214.10(P:GND) IC215.10(P:GND) IC216.10(GND) IC217.10(P:GND) IC218.7(P:GND) IC219.7(P:GND) IC220.7(P:GND) IC221.7(P:GND) IC222.8(GND) IC223.7(P:GND) IC224.7(P:GND) IC225.7(P:GND) IC226.8(GND) IC227.7(P:GND) IC228.7(P:GND) IC229.10(P:GND) IC230.10(P:GND) IC231.10(P:GND) IC232.10(P:GND) IC233.10(GND) IC234.10(GND) IC235.10(P:GND) IC236.10(P:GND) IC237.10(P:GND) IC238.10(P:GND) IC239.10(GND) IC240.10(GND) IC241.7(P:GND) IC242.7(P:GND) IC243.7(P:GND) IC244.10(P:GND) IC245.10(P:GND) IC246.10(P:GND) IC247.10(P:GND) IC248.8(GND) IC249.8(GND) IC250.7(P:GND)
VCC: IC1.20(VCC) IC2.20(P:VCC) IC3.20(P:VCC) IC4.20(VCC) IC5.20(VCC) IC6.20(VCC) IC7.20(VCC) IC8.20(P:VCC) IC9.20(P:VCC) IC10.20(P:VCC) IC11.20(P:VCC) IC12.20(P:VCC) IC13.20(P:VCC) IC14.24(VCC) IC15.24(VCC) IC16.20(VCC) IC17.20(VCC) IC18.14(P:VCC) IC19.20(P:VCC) IC20.20(VCC) IC21.20(VCC) IC22.16(VCC) IC23.16(VCC) IC24.20(P:VCC) IC25.20(P:VCC) IC26.20(P:VCC) IC27.20(P:VCC) IC28.20(P:VCC) IC29.20(P:VCC) IC30.20(P:VCC) IC31.20(P:VCC) IC32.20(VCC) IC33.20(VCC) IC34.16(VCC) IC35.16(VCC) IC36.16(VCC) IC37.16(VCC) IC38.16(VCC) IC39.14(P:VCC) IC40.16(VCC) IC41.16(VCC) IC42.14(P:VCC) IC43.14(P:VCC) IC44.14(P:VCC) IC45.14(P:VCC) IC46.20(VCC) IC47.16(VCC) IC48.20(VCC) IC49.16(VCC) IC50.16(VCC) IC51.16(VCC) IC52.16(VCC) IC53.16(VCC) IC54.14(P:VCC) IC55.16(VCC) IC56.16(VCC) IC57.14(P:VCC) IC58.14(P:VCC) IC59.16(VCC) IC60.20(VCC) IC61.20(VCC) IC62.20(VCC) IC63.16(VCC) IC64.14(P:VCC) IC65.14(P:VCC) IC66.14(P:VCC) IC67.14(P:VCC) IC68.16(VCC) IC69.20(P:VCC) IC70.20(P:VCC) IC71.20(P:VCC) IC72.14(P:VCC) IC73.16(VCC) IC74.14(P:VCC) IC75.20(VCC) IC76.20(VCC) IC77.20(VCC) IC78.20(VCC) IC79.20(VCC) IC80.14(P:VCC) IC81.14(P:VCC) IC82.20(VCC) IC83.14(P:VCC) IC84.14(P:VCC) IC85.14(P:VCC) IC86.20(VCC) IC87.16(P:VCC) IC88.20(VCC) IC89.20(P:VCC) IC90.20(P:VCC) IC91.20(P:VCC) IC92.20(P:VCC) IC93.20(VCC) IC94.16(VCC) IC95.16(VCC) IC96.16(VCC) IC97.16(VCC) IC98.20(VCC) IC99.20(VCC) IC100.20(VCC) IC101.20(VCC) IC102.20(P:VCC) IC103.20(VCC) IC104.20(VCC) IC105.20(P:VCC) IC106.20(P:VCC) IC107.20(P:VCC) IC108.20(P:VCC) IC109.20(P:VCC) IC110.20(P:VCC) IC111.20(P:VCC) IC112.20(P:VCC) IC113.20(P:VCC) IC114.20(P:VCC) IC115.20(P:VCC) IC116.20(P:VCC) IC117.20(P:VCC) IC118.20(VCC) IC119.16(VCC) IC120.14(P:VCC) IC121.16(VCC) IC122.20(P:VCC) IC123.20(VCC) IC124.20(P:VCC) IC125.20(P:VCC) IC126.20(VCC) IC127.14(P:VCC) IC128.16(VCC) IC129.20(P:VCC) IC130.14(P:VCC) IC131.14(P:VCC) IC132.14(P:VCC) IC133.14(P:VCC) IC134.20(VCC) IC135.20(VCC) IC136.20(VCC) IC137.20(VCC) IC138.14(P:VCC) IC139.16(VCC) IC140.20(VCC) IC141.14(P:VCC) IC142.16(VCC) IC143.14(P:VCC) IC144.16(VCC) IC145.20(P:VCC) IC146.20(P:VCC) IC147.14(P:VCC) IC148.14(P:VCC) IC149.14(P:VCC) IC150.14(P:VCC) IC151.14(P:VCC) IC152.14(P:VCC) IC153.20(VCC) IC154.20(P:VCC) IC155.20(P:VCC) IC156.20(P:VCC) IC157.14(P:VCC) IC158.14(P:VCC) IC159.20(P:VCC) IC160.20(P:VCC) IC161.20(P:VCC) IC162.20(VCC) IC163.14(P:VCC) IC164.14(P:VCC) IC165.20(VCC) IC166.20(VCC) IC167.16(VCC) IC168.14(P:VCC) IC169.16(VCC) IC170.14(P:VCC) IC171.16(VCC) IC172.16(VCC) IC173.16(VCC) IC174.14(P:VCC) IC175.14(P:VCC) IC176.20(P:VCC) IC177.14(P:VCC) IC178.20(P:VCC) IC179.20(P:VCC) IC180.20(VCC) IC181.20(P:VCC) IC182.20(P:VCC) IC183.20(P:VCC) IC184.20(VCC) IC185.20(VCC) IC186.20(P:VCC) IC187.14(P:VCC) IC188.14(P:VCC) IC189.20(VCC) IC190.14(P:VCC) IC191.14(P:VCC) IC192.14(P:VCC) IC193.14(P:VCC) IC194.14(P:VCC) IC195.20(P:VCC) IC196.20(P:VCC) IC197.14(P:VCC) IC198.14(P:VCC) IC199.14(P:VCC) IC200.14(P:VCC) IC201.14(P:VCC) IC202.14(P:VCC) IC203.14(P:VCC) IC204.14(P:VCC) IC205.14(P:VCC) IC206.14(P:VCC) IC207.14(P:VCC) IC208.14(P:VCC) IC209.14(P:VCC) IC210.16(VCC) IC211.20(P:VCC) IC212.20(P:VCC) IC213.20(P:VCC) IC214.20(P:VCC) IC215.20(P:VCC) IC216.20(VCC) IC217.20(P:VCC) IC218.14(P:VCC) IC219.14(P:VCC) IC220.14(P:VCC) IC221.14(P:VCC) IC222.16(VCC) IC223.14(P:VCC) IC224.14(P:VCC) IC225.14(P:VCC) IC226.16(VCC) IC227.14(P:VCC) IC228.14(P:VCC) IC229.20(P:VCC) IC230.20(P:VCC) IC231.20(P:VCC) IC232.20(P:VCC) IC233.20(VCC) IC234.20(VCC) IC235.20(P:VCC) IC236.20(P:VCC) IC237.20(P:VCC) IC238.20(P:VCC) IC239.20(VCC) IC240.20(VCC) IC241.14(P:VCC) IC242.14(P:VCC) IC243.14(P:VCC) IC244.20(P:VCC) IC245.20(P:VCC) IC246.20(P:VCC) IC247.20(P:VCC) IC248.16(VCC) IC249.16(VCC) IC250.14(P:VCC)

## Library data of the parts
IC1 IC4-IC7 IC16 IC17 IC21 IC48 IC82 IC86 IC88 IC93 IC98-IC101 IC123 IC153 IC180 IC184 IC185 IC189 IC216 IC233 IC234 IC239 IC240 = 74xx-us:74*377: Octal D type FLIP FLOP, enable
IC2 IC3 IC8-IC13 IC24-IC31 IC69-IC71 IC102 IC105-IC117 IC122 IC124 IC125 IC129 IC145 IC146 IC154 IC155 IC176 IC178 IC179 IC181-IC183 IC186 IC195 IC196 IC215 IC244-IC247 = 74xx-us:74*244: Octal BUFFER and LINE DRIVER, 3-state; MF: TEXAS INSTRUMENTS; MPN: SN74LS244N; OC_FARNELL: 1739688
IC14 IC15 = 74xx-us:74*181: ARITHMETIC LOGIC UNIT function generator; OC_FARNELL: unknown
IC18 IC66 IC67 IC81 IC147 IC170 IC250 = 74xx-us:74*32: Quad 2-input OR gate; MF: TEXAS INSTRUMENTS; MPN: SN7432N; OC_FARNELL: 1607803
IC19 IC89-IC92 IC211-IC214 IC217 IC229-IC232 IC235-IC238 = 74xx-us:74*244: Octal BUFFER and LINE DRIVER, 3-state; OC_FARNELL: unknown
IC20 IC32 IC33 IC60-IC62 IC75-IC79 IC134-IC137 = 74xx-us:74*273: Octal D type FLIP FLOP, clear; OC_FARNELL: unknown
IC22 IC23 IC47 IC94-IC97 IC119 IC121 IC167 IC210 = 74xx-us:74*157: Quadruple 2-line to 1-line data SELECTOR/MULTIPLEXER; OC_FARNELL: unknown
IC34-IC38 IC40 IC41 IC56 IC142 = 74xx-us:74*153: Dual 4-line to 1-line data SELECTOR/MULTIPLEXER; OC_FARNELL: unknown
IC39 IC42 IC45 IC120 IC127 IC133 IC138 IC143 IC207 IC208 IC218-IC220 IC223-IC225 = 74xx-us:74*08: Quad 2-input AND gate; OC_FARNELL: unknown
IC43 IC54 IC57 IC65 IC83 IC84 IC132 IC141 IC150 IC151 IC157 IC158 IC198 = 74xx-us:74*04: Hex INVERTER; OC_FARNELL: unknown
IC44 = 74xx-us:74*74: Dual D type positive edge triggered FLIP FLOP, preset and clear; OC_FARNELL: unknown
IC46 IC126 = 74xx-us:74*377: Octal D type FLIP FLOP, enable; OC_FARNELL: unknown
IC49 IC55 IC59 IC63 IC68 IC73 IC169 IC171-IC173 = 74xx-us:74*257: Quadruple 2-to 1 line data SELECTOR/MULTIPLEXER; OC_FARNELL: unknown
IC50-IC53 = 74xx-us:74*283: 4-bit binary FULL ADDER, fast carry; OC_FARNELL: unknown
IC58 IC72 IC74 IC80 IC130 IC175 IC177 IC192-IC194 IC200 IC209 = 74xx-us:74*86: Quad 2-input EXCLUSIV-OR (XOR) gate; OC_FARNELL: unknown
IC64 IC131 = 74xx-us:74*20: Dual 4-input NAND gate; OC_FARNELL: unknown
IC85 = 74xx-us:74*10: Triple 3-input NAND gate
IC87 = 74xx-us:74*279: Quadruple S-R LATCH; OC_FARNELL: unknown
IC103 IC104 IC118 IC140 IC165 IC166 = 74xx-us:74*541: Octal BUFFER and LINE DRIVER, 3-state; OC_FARNELL: unknown
IC128 IC144 IC248 IC249 = 74xx-us:74*173: 4-bit D type REGISTER, 3-state
IC139 = 74xx-us:74*173: 4-bit D type REGISTER, 3-state; OC_FARNELL: unknown
IC148 IC149 IC152 = 74xx-us:74*04: Hex INVERTER
IC156 IC159-IC161 = 74xx-us:74*244: Octal BUFFER and LINE DRIVER, 3-state
IC162 = 74xx-us:74*273: Octal D type FLIP FLOP, clear
IC163 IC164 IC168 IC174 IC187 IC188 IC221 = 74xx-us:74*74: Dual D type positive edge triggered FLIP FLOP, preset and clear
IC190 IC191 IC201-IC203 IC205 IC206 IC227 IC228 IC241-IC243 = 74xx-us:74*00: Quad 2-input NAND gate
IC197 IC199 = 74xx-us:74*260: Dual 5-input positive NOR gate; OC_FARNELL: unknown
IC204 = 74xx-us:74*11: Triple 3-input AND gate
IC222 = 74xx-us:74*138: 3-line to 8-line DECODER/DEMULTIPLEXER
IC226 = 74xx-us:74*148: 10-line to 4-line and 8-line to 3-line PRIORITY ENCODER
R1-R3 R9 = rcl:R-US_: RESISTOR, American symbol; OC_FARNELL: unknown
R4-R8 R10 = resistor-bourns:4816P-T01: BOURNS RESISTOR NETWORK; MF: BOURNS; MPN: 4816P-T01-104LF; OC_FARNELL: 9357483; OC_NEWARK: 33K0707
S1 S2 S4 = switch:TL36PO: TINY SWITCH ON - ON Source: http://www2.produktinfo.conrad.com/datenblaetter/700000-724999/705152-da-01-de-Subminiaturschalter_TL_36YO.pdf; OC_FARNELL: unknown
S3 = switch:50-1POLE22,5: SERIES 50 Single-Deck Rotary Switches one pole 22.5° Source: www.grayhill.com .. J-15-21.pdf
SW1 SW2 = special:SW_DIP-8: DIP SWITCH; OC_FARNELL: unknown
SW3 = special:SW-C10: SWITCH 10-step rotary switch; OC_FARNELL: unknown
U$1-U$12 = atmel_28c:AT28C256-28DIP: IC EEPROM 256KBIT 150NS 28DIP; OC_FARNELL: unknown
